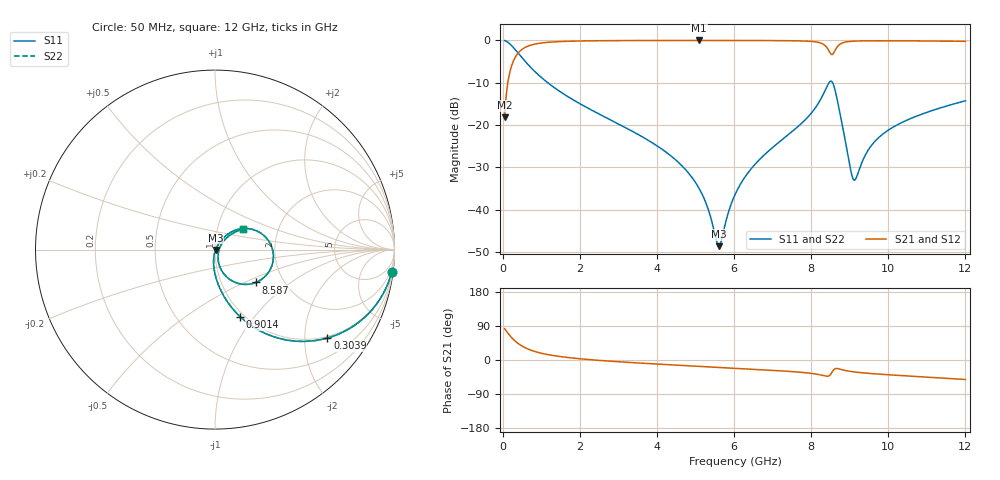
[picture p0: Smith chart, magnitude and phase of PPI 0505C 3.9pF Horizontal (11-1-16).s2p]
# MHz S MA R 50
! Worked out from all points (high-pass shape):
!   1601 points, 50 MHz to 12 GHz, reference 50 ohm
!   highest |S21| = -0.03 dB at 5.091 GHz (marker M1); lowest = -18.2 dB at 50 MHz (marker M2)
!   |S21| within 3 dB of the highest: 398.8 MHz to 8.495 GHz (8.097 GHz wide, 182 % of centre); 8.58 GHz to end of sweep
!   lowest |S11| = -48.6 dB at 5.607 GHz (marker M3), VSWR 1.01, Z = 50.3 - j0.131 ohm
!   |S11| at or under -10 dB: 1.166 GHz to 8.462 GHz (7.296 GHz wide, 152 % of centre); 8.556 GHz to end of sweep
!   |S22| runs from -48.6 to -0.1 dB; largest |S21 - S12| = 0
!   S11 on the Smith chart (normalised r, x): 50 MHz: 1, -16; 303.9 MHz: 0.95, -2.58; 901.4 MHz: 0.96, -0.85; 8.587 GHz: 1.45, -0.58; 12 GHz: 1.33, +0.32
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50  0.9923 -7.3  0.1234 82.7  0.1234 82.7  0.9923 -7.3
169.5  0.9212 -23.5  0.3887 66.5  0.3887 66.5  0.9212 -23.5
303.9375  0.7967 -38.2  0.6037 51.8  0.6037 51.8  0.7967 -38.2
565.3438  0.5761 -56.7  0.8163 33.2  0.8163 33.2  0.5761 -56.7
901.4375  0.4003 -69.4  0.915 20.4  0.915 20.4  0.4003 -69.4
2044.156  0.1738 -86.5  0.9826 2.9  0.9826 2.9  0.1738 -86.5
4038.312  0.05525 -97.9  0.9953 -10.9  0.9953 -10.9  0.05525 -97.9
4665.688  0.03232 -98.8  0.996 -14.4  0.996 -14.4  0.03232 -98.8
5091.406  0.01787 -95.7  0.9961 -16.7  0.9961 -16.7  0.01787 -95.7
5606.75  0.003695 -20.7  0.9959 -19.4  0.9959 -19.4  0.003695 -20.7
6025  0.01501 52.8  0.9955 -21.7  0.9955 -21.7  0.01501 52.8
6585.156  0.0359 57.8  0.9943 -24.8  0.9943 -24.8  0.0359 57.8
8019.156  0.1406 46.2  0.9696 -35.5  0.9696 -35.5  0.1406 46.2
8370.188  0.2615 22.4  0.8597 -42.4  0.8597 -42.4  0.2615 22.4
8489.688  0.3268 -5.5  0.7119 -39.6  0.7119 -39.6  0.3268 -5.5
8586.781  0.292 -38.8  0.713 -25.6  0.713 -25.6  0.292 -38.8
8766.031  0.1242 -72.3  0.9114 -24.7  0.9114 -24.7  0.1242 -72.3
9019.969  0.03018 -53.4  0.9716 -30.1  0.9716 -30.1  0.03018 -53.4
9109.594  0.02229 -18.8  0.9777 -31.4  0.9777 -31.4  0.02229 -18.8
9535.312  0.05501 42.5  0.9866 -35.6  0.9866 -35.6  0.05501 42.5
10013.31  0.08758 45.4  0.9871 -39.0  0.9871 -39.0  0.08758 45.4
12000  0.1931 36.4  0.973 -51.4  0.973 -51.4  0.1931 36.4
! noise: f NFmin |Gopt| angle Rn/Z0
50  0.0005905  0.9199  2.021  0.001629
1372  0.004935  0.7288  5.623  0.003613
2701  0.00805  0.6821  9.969  0.004869
4031  0.01092  0.6572  14.34  0.005987
5360  0.01389  0.6466  18.66  0.007266
6682  0.01795  0.6594  22.88  0.009685
8012  0.03958  0.8012  27.31  0.039
9341  0.03581  0.7536  31.77  0.02719
1.067e+04  0.02795  0.6628  35.5  0.01446
1.2e+04  0.02969  0.6511  39.23  0.01443
